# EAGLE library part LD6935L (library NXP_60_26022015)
Dual low-dropout regulators, high PSRR, 300 mA The LD6935 series consists of small-size dual Low DropOut regulators (LDO). Each device delivers two times 300 mA with a typical voltage drop of 240 mV at 300 mA for each LDO. Each device offers two individual fixed nominal output voltages (VO(nom)) from 1.2 V to 3.6 V. The LDO has an integrated Soft start to control the inrush current during start-up. The output states when disabled can be high-ohmic 3-state or auto discharge. Optionally a delayed output circuit is available for the second output. The devices are available in DFN1612-8 (SOT1225) plastic package with a height of 0.4 mm. AAL Eindhoven MK
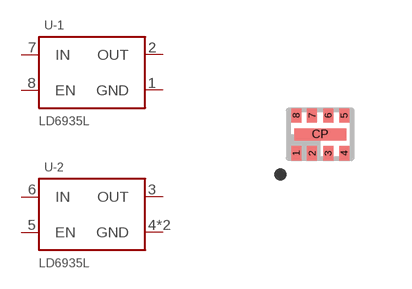
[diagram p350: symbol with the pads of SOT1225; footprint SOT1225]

Designator prefix U; gates -1=LD680X -2=LD680X

## LD6935L/1828P (OUT1: 1V8; OUT2: 2V8; OUTPUT: Pull Down), LD6935L/2828H (OUT1: 2V8; OUT2: 2V8; OUTPUT: High Ohmic), LD6935L/2828P (OUT1: 2V8; OUT2: 2V8; OUTPUT: Pull Down), LD6935L/3118PD (MISC: Delay Circuit; OUT1: 3V1; OUT2: 1V8; OUTPUT: Pull Down), LD6935L/3318H (OUT1: 3V3; OUT2: 1V8; OUTPUT: High Ohmic), LD6935L/3318P (OUT1: 3V3; OUT2: 1V8; OUTPUT: Pull Down), LD6935L/3328P (OUT1: 3V3; OUT2: 2V8; OUTPUT: Pull Down), LD6935L/3333P (OUT1: 3V3; OUT2: 3V3; OUTPUT: Pull Down)  [SOT1225]
1  -1:GND  pwr
2  -1:OUT  pas
3  -2:OUT  pas
4  -2:GND  pwr
5  -2:EN  in
6  -2:IN  pas
7  -1:IN  pas
8  -1:EN  in
CP  -2:GND  pwr

## Footprint SOT1225 (pad centres in mm)
SOT1225 DFN1612-8: plastic extremely thin small outline package; no leads; 8 terminals; body 1.6 x 1.2 x 0.4 mm JEDEC: IEC: -- JEITA: --date: 2013-06-28
smd 0.25 x 0.35: 1 -0.6,-0.475; 2 -0.2,-0.475; 3 0.2,-0.475; 4 0.6,-0.475; 5 0.6,0.475; 6 0.2,0.475; 7 -0.2,0.475; 8 -0.6,0.475
smd 1.3 x 0.3: CP 0,0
